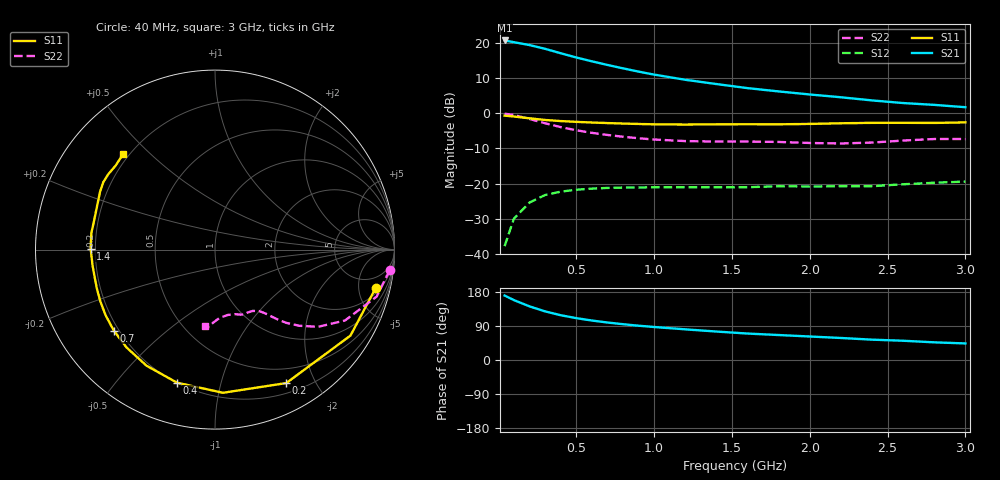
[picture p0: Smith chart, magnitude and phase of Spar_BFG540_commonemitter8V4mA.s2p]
! Filename:  BFG540G.S2P  Version:  3.0
! NXP part #: BFG540  Date: Feb 1992
! Bias condition: Vce=8V, Ic=4mA
! IN LINE PINNING: same data as with cross emitter pinning.
#  MHz  S  MA  R  50
! Freq  S11  S21  S12  S22  !GUM [dB]
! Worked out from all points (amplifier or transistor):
!   21 points, 40 MHz to 3 GHz, reference 50 ohm
!   highest |S21| = 20.6 dB at 40 MHz (marker M1)
!   |S21| within 3 dB of that: start of sweep to 350.3 MHz
!   unconditionally stable (mu >= 1): 1.791 GHz to end of sweep
!   at 300 MHz: K = 0.17, MSG = 20.7 dB, |S12| = -23.2 dB
!   at 1 GHz: K = 0.59, MSG = 16.0 dB, |S12| = -21.0 dB
!   at 3 GHz: K = 1.33, MAG = 7.1 dB, |S12| = -19.4 dB
!   S11 on the Smith chart (normalised r, x): 40 MHz: 2.73, -7.62; 200 MHz: 0.32, -1.62; 400 MHz: 0.20, -0.74; 700 MHz: 0.18, -0.34; 1.4 GHz: 0.18, +0.00; 3 GHz: 0.18, +0.41
40  0.921 -13.3  10.7 170.2  0.013 81.1  0.98 -6.7
100  0.894 -32.4  10.11 158.0  0.032 70.9  0.938 -16.2
200  0.843 -61.9  9.196 141.5  0.054 56.4  0.825 -28.6
300  0.799 -86.8  8.142 128.3  0.069 46.1  0.718 -36.8
400  0.771 -105.9  7.047 118.2  0.077 39.3  0.633 -42.1
500  0.751 -120.5  6.137 110.5  0.082 34.5  0.571 -45.7
600  0.735 -132.1  5.419 104.2  0.085 31.7  0.525 -48.0
700  0.722 -141.3  4.813 98.9  0.087 29.5  0.49 -49.7
800  0.711 -149.0  4.306 94.5  0.088 27.8  0.462 -51.2
900  0.701 -155.7  3.871 90.5  0.088 27.3  0.44 -52.7
1000  0.693 -161.9  3.511 87.1  0.089 26.9  0.422 -54.3
1200  0.688 -172.3  2.966 80.9  0.089 27.0  0.401 -58.4
1400  0.693 179.5  2.58 75.1  0.089 27.4  0.395 -62.6
1600  0.695 172.5  2.258 69.8  0.089 30.5  0.395 -65.8
1800  0.693 165.7  2.028 65.9  0.092 32.4  0.39 -68.4
2000  0.702 158.9  1.834 62.0  0.091 35.5  0.377 -72.6
2200  0.717 153.3  1.676 58.1  0.092 38.5  0.371 -79.1
2400  0.727 148.9  1.512 53.7  0.092 42.3  0.382 -86.3
2600  0.728 144.8  1.387 50.8  0.098 45.5  0.408 -91.6
2800  0.725 139.7  1.307 46.6  0.103 47.4  0.429 -94.4
3000  0.738 134.1  1.211 43.7  0.107 51.7  0.429 -97.1
